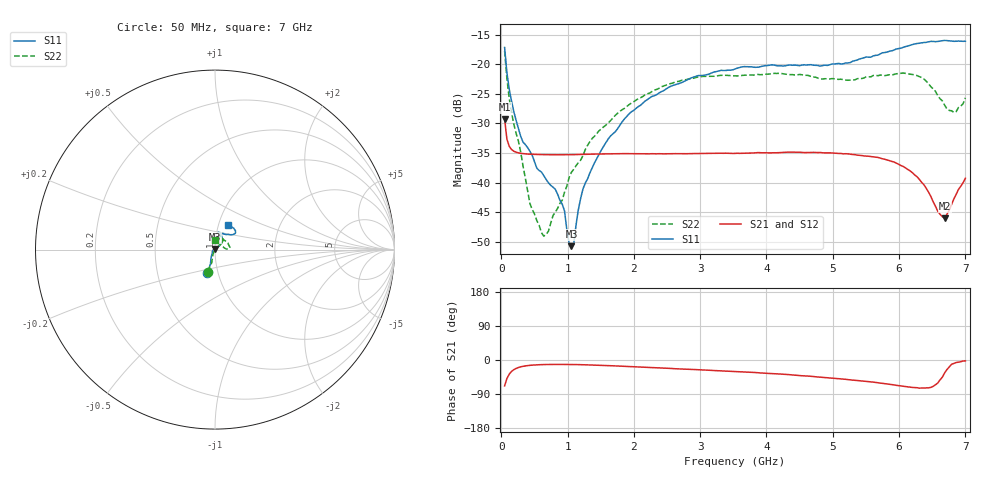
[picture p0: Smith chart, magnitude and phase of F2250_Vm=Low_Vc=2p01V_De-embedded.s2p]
! Integrated Device Technology
! Corporate Headquarters
! 6024 Silver Creek Valley Road
! San Jose, CA 95138  USA
! Phone:  1-408-284-8200
! Toll Free:  1-800-223-1366
! Webpage:  http://www.idt.com/
! Timing and RF Division
! 515 Groton Road, Suite 102
! Westford, MA 01886-6024
! Device:  F2250
! Description: Voltage Variable RF Attenuator
! Frequency:  50.0 -  6000.00 MHz
! Package:  3x3 mm Thin QFN Plastic Package: 16 pin
! Ports:  2 RF, 3 DC
!  Pin  1  = GND
!  Pin  2  = NC
!  Pin  3  = RF1  = Port 1
!  Pin  4  = NC
!  Pin  5  = GND
!  Pin  6  = GND
!  Pin  7  = GND
!  Pin  8  = GND
!  Pin  9  = NC
!  Pin 10  = RF2  = Port 2
!  Pin 11  = NC
!  Pin 12  = GND
!  Pin 13  = GND
!  Pin 14  = VCNTRL
!  Pin 15  = VDD
!  Pin 16  = VMODE
! Vcntrl:  2.010 Volts
! Vmode:  +0.000 Volts
! Vdd:  +3.30  Volts
! Current:  1.181 mA
! Data:  The device was measured on a the F2250 evaluation board which has
!  individual transmission lines to the RF pins.  Data was collected
!  using a calibrated network analyzer.  The evaluation board was
!  de-embedded using a TRL calibration technique.
!  The reference plane is the edge of the package pin.
! Misc:  SN 10
!  Action Tracker AT0258
! Date Measured:  2014-11-26
! Date:  2015-10-15  MJV
! Note:
!  Integrated Device Technology supplies this data as a sample of measured
!  data at the package pin for this product.  Your particular data for this
!  product may vary.
!  Data was taken at 25 degrees C.
!  Integrated Device Technology reserves the right to change this data at anytime.
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# GHz S dB R 50
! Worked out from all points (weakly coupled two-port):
!   201 points, 50 MHz to 7 GHz, reference 50 ohm
!   highest |S21| = -29.28 dB at 50 MHz (marker M1); lowest = -46.0 dB at 6.687 GHz (marker M2)
!   lowest |S11| = -50.7 dB at 1.058 GHz (marker M3), VSWR 1.01, Z = 49.8 + j0.244 ohm
!   |S11| at or under -10 dB: start of sweep to end of sweep
!   |S22| runs from -49.0 to -17.8 dB; largest |S21 - S12| = 6.4e-05
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0.05  -17.18 -108.6  -29.28 -68.3  -29.27 -68.3  -17.78 -108.5
0.08475  -21.44 -107.4  -32.66 -49.0  -32.66 -49.0  -22.45 -104.1
0.1195  -24.19 -111.7  -33.87 -37.4  -33.87 -37.4  -25.76 -106.8
0.29325  -32.21 -127.6  -35.06 -18.0  -35.05 -18.0  -34.87 -113.6
0.43225  -34.72 -144.5  -35.20 -14.1  -35.20 -14.1  -43.56 -141.6
0.606  -38.21 -160.9  -35.27 -12.2  -35.27 -12.2  -48.46 158.9
0.71025  -40.02 -168.2  -35.29 -11.8  -35.29 -11.8  -48.24 114.4
0.91875  -43.64 158.0  -35.30 -11.7  -35.30 -11.7  -42.99 77.9
1.023  -50.23 143.2  -35.29 -11.8  -35.29 -11.8  -39.15 68.0
1.05775  -50.74 122.4  -35.29 -11.9  -35.28 -11.9  -38.26 65.3
1.0925  -50.44 88.6  -35.28 -12.0  -35.28 -11.9  -37.75 61.4
1.162  -44.60 56.4  -35.26 -12.2  -35.26 -12.2  -36.62 52.8
1.2315  -41.09 43.7  -35.23 -12.4  -35.23 -12.4  -35.44 47.3
1.6485  -32.12 41.8  -35.15 -15.1  -35.15 -15.1  -29.52 45.6
2.37825  -24.87 47.3  -35.12 -20.9  -35.13 -20.9  -24.08 47.0
3.525  -20.81 72.5  -35.07 -30.5  -35.07 -30.5  -21.98 69.6
4.7065  -20.17 72.4  -34.89 -43.6  -34.89 -43.6  -22.16 69.3
5.85325  -17.82 40.4  -36.29 -64.1  -36.29 -64.1  -21.78 17.7
6.33975  -16.40 40.9  -39.95 -74.0  -39.95 -74.1  -22.26 3.5
6.68725  -15.99 48.8  -46.01 -34.1  -45.99 -33.6  -26.92 23.8
6.861  -16.13 55.1  -41.99 -6.7  -41.96 -6.7  -28.02 58.6
7  -16.12 63.2  -39.27 -2.5  -39.22 -2.5  -25.68 87.1
